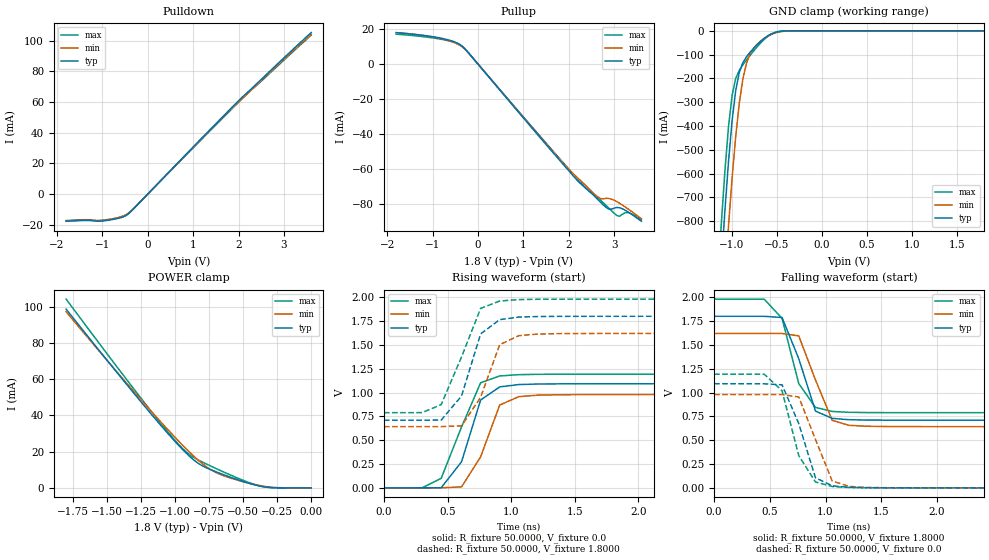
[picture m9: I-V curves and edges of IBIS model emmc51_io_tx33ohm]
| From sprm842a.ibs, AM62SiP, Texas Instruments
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|4LPDDR4X ********** End LPDDR4X Models *********************************
|1EMMC ********************* Start EMMC *********************************
|   Model emmc51_io_tx33ohm
[Model]  emmc51_io_tx33ohm
Model_type I/O
Polarity   Non-Inverting
Enable   Active-High
Vinl =   0.6300V
Vinh =   1.1700V
Vmeas =  0.2000V
Cref =   0.5000pF
Rref =   50.0000
Vref =   0.2000V
C_comp   2.0000pF   2.0000pF   2.0000pF
[Temperature Range]   25.0000   0.1250k   -40.0000
[Voltage Range]   1.8000V   1.6200V   1.9800V
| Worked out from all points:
|   slope of the pulldown table from 0 to 0.27 V, typ, clamps not added: 32.5 ohm
|   slope of the pullup table from 0 to 0.27 V, typ, clamps not added: 32.4 ohm
|   GND clamp passes 1 mA (typ) near -0.43 V on its own axis
|   POWER clamp passes 1 mA (typ) near -0.38 V on its own axis
|   rising waveform, R_fixture 50.0000, V_fixture 0.0: 20-80 % time 171ps typ, 188ps min, 221ps max; typ from 0 V to 1.09 V
|   rising waveform, R_fixture 50.0000, V_fixture 1.8000: 20-80 % time 165ps typ, 185ps min, 219ps max; typ from 0.71 V to 1.8 V
|   falling waveform, R_fixture 50.0000, V_fixture 1.8000: 20-80 % time 195ps typ, 199ps min, 182ps max; typ from 1.8 V to 0.71 V
|   falling waveform, R_fixture 50.0000, V_fixture 0.0: 20-80 % time 194ps typ, 200ps min, 190ps max; typ from 1.09 V to 0 V
[Pulldown]
|Voltage   I(typ)   I(min)   I(max)
-1.8V     -17.77mA   -17.5mA    -17.3mA
-1.38V    -17.23mA   -16.98mA   -16.74mA
-1.14V    -17.67mA   -17.21mA   -17.33mA
-960mV    -17.44mA   -17.04mA   -16.98mA
-600mV    -15.45mA   -14.88mA   -15.19mA
-480mV    -13.99mA   -13.43mA   -13.86mA
-420mV    -12.72mA   -12.3mA    -12.58mA
-300mV    -9.232mA   -9.12mA    -9.074mA
1.62V     49.45mA    48.96mA    48.64mA
2.22V     66.89mA    66.08mA    66.25mA
3.6V      105.2mA    104mA      103.6mA
[Pullup]
|Voltage   I(typ)   I(min)   I(max)
-1.8V     17.89mA    17.97mA    17.07mA
-840mV    14.89mA    14.66mA    14.29mA
-360mV    10.5mA     10.03mA    10.37mA
-180mV    5.562mA    5.485mA    5.464mA
1.92V     -58.65mA   -57.94mA   -57.69mA
2.4V      -71.57mA   -70.22mA   -71.62mA
2.7V      -79mA      -76.96mA   -77.88mA
2.88V     -82.97mA   -76.88mA   -82.37mA
3.06V     -82.05mA   -78.72mA   -86.66mA
3.12V     -82.21mA   -79.64mA   -87.05mA
3.3V      -84.5mA    -82.79mA   -84.94mA
3.6V      -89.96mA   -88.47mA   -89.15mA
[GND_clamp]
|Voltage   I(typ)   I(min)   I(max)
-1.8V     -6.702A    -6.906A    -6.586A
-1.12V    -991.1mA   -1.287A    -813.9mA
-1.08V    -758.6mA   -1.044A    -591.9mA
-1.04V    -552.1mA   -821.7mA   -405.1mA
-1V       -379.5mA   -621.1mA   -272.1mA
-960mV    -252.2mA   -446.8mA   -200.8mA
-920mV    -175.1mA   -305.6mA   -166.2mA
-880mV    -134mA     -202.7mA   -143.1mA
-800mV    -90.55mA   -97.27mA   -103.4mA
-600mV    -20.52mA   -21.87mA   -22.63mA
-400mV    -332.1uA   -1.109mA   -151.2uA
1.8V      231.4nA    26.73uA    254.2nA
[POWER_clamp]
|Voltage   I(typ)   I(min)   I(max)
-1.8V     98.61mA    97.2mA     104.1mA
-1.44V    64.88mA    65.13mA    68.09mA
-1.16V    39.38mA    40.99mA    40.81mA
-1V       25.58mA    27.85mA    26.18mA
-900mV    17.84mA    20.17mA    18.67mA
-820mV    13.08mA    14.63mA    15mA
-740mV    10.1mA     10.15mA    12.1mA
-660mV    7.73mA     7.169mA    9.318mA
-560mV    4.993mA    4.669mA    6.008mA
-440mV    2.128mA    2.259mA    2.491mA
-340mV    491.7uA    786.4uA    470uA
0V        231.4nA    1.21uA     740.9nA
[Ramp]
| variable   typ   min   max
dV/dt_r  0.6552/0.1693n   0.5872/0.1882n   0.7156/0.2135n
dV/dt_f  0.6542/0.1954n   0.5867/0.1991n   0.7146/0.1819n
R_load = 50.0000
[Rising Waveform]
R_fixture= 50.0000
V_fixture= 0.0
V_fixture_min= 0.0
V_fixture_max= 0.0
|time   V(typ)   V(min)   V(max)
0s        1.212uV    12.34uV    2.539uV
300ps     171.4uV    34.27uV    609.5uV
450ps     1.377mV    378.4uV    100mV
610ps     273.5mV    10.71mV    638.8mV
760ps     921.7mV    325.6mV    1.102V
910ps     1.059V     868.8mV    1.174V
1.06ns    1.084V     956.8mV    1.188V
1.21ns    1.089V     972.7mV    1.191V
1.82ns    1.092V     978.6mV    1.193V
15ns      1.092V     978.7mV    1.193V
[Rising Waveform]
R_fixture= 50.0000
V_fixture= 1.8000
V_fixture_min= 1.6200
V_fixture_max= 1.9800
|time   V(typ)   V(min)   V(max)
0s        709.7mV    642.1mV    789mV
300ps     709.8mV    642.2mV    789.5mV
450ps     711mV      642.5mV    873.4mV
610ps     964.3mV    650.9mV    1.374V
760ps     1.615V     950.4mV    1.883V
910ps     1.765V     1.502V     1.96V
1.06ns    1.792V     1.597V     1.975V
1.21ns    1.797V     1.614V     1.978V
1.67ns    1.8V       1.62V      1.98V
15ns      1.8V       1.62V      1.98V
[Falling Waveform]
R_fixture= 50.0000
V_fixture= 1.8000
V_fixture_min= 1.6200
V_fixture_max= 1.9800
|time   V(typ)   V(min)   V(max)
0s        1.8V       1.62V      1.98V
450ps     1.8V       1.62V      1.979V
610ps     1.787V     1.62V      1.778V
760ps     1.355V     1.594V     1.093V
910ps     805.5mV    1.132V     843.9mV
1.06ns    729.2mV    708.7mV    801.8mV
1.21ns    715mV      656.4mV    792.5mV
1.36ns    711.4mV    646.5mV    790.1mV
1.67ns    709.9mV    642.8mV    789.1mV
15ns      709.7mV    642.1mV    789mV
[Falling Waveform]
R_fixture= 50.0000
V_fixture= 0.0
V_fixture_min= 0.0
V_fixture_max= 0.0
|time   V(typ)   V(min)   V(max)
0s        1.092V     978.7mV    1.193V
450ps     1.092V     978.7mV    1.192V
610ps     1.081V     978.4mV    1.019V
760ps     673.5mV    953.5mV    338.3mV
910ps     105.5mV    508mV      61.68mV
1.06ns    21.58mV    72.31mV    14.28mV
1.21ns    5.855mV    15.44mV    3.973mV
1.36ns    1.947mV    4.655mV    1.26mV
1.67ns    295.8uV    762.5uV    167.6uV
15ns      1.298uV    12.34uV    2.401uV
